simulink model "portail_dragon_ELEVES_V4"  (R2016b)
settings: Solver=VariableStepAuto  StartTime=0.0  StopTime=inf  FixedStep=1e-3  RelTol=1e-3  EnableMultiTasking=on
libraries: fl_lib x6, nesl_utility x5, simulink x2, realtime_pacer_lib x1

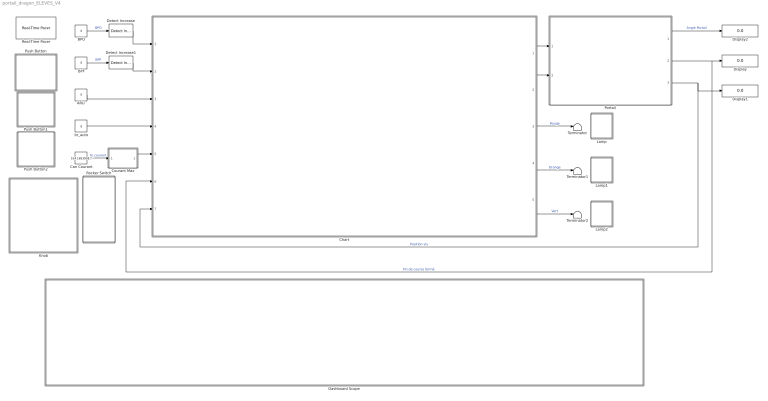
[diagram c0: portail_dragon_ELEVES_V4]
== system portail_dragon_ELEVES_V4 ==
  "ARU " : Constant  Value=0
  BPF : Constant  Value=0
  BPO : Constant  Value=0
  Can Courant : Constant  Value=514.18539581299
  Chart : Stateflow chart  TreatAsAtomicUnit=on
  Courant Max : MATLAB Function  TreatAsAtomicUnit=on
  Dashboard Scope : Subsystem  DialogController=hmiCreateDDGDialog  IsWebBlock=on
  Detect Increase : simulink/Logic and Bit Operations/Detect Increase  vinit=0.0  OutDataTypeStr=boolean
  Detect Increase1 : simulink/Logic and Bit Operations/Detect Increase  vinit=0.0  OutDataTypeStr=boolean
  Display : Display
  Display1 : Display
  Display2 : Display
  Knob : Subsystem  DialogController=hmiCreateDDGDialog  IsWebBlock=on
  Lamp : Subsystem  DialogController=hmiCreateDDGDialog  IsWebBlock=on
  Lamp1 : Subsystem  DialogController=hmiCreateDDGDialog  IsWebBlock=on
  Lamp2 : Subsystem  DialogController=hmiCreateDDGDialog  IsWebBlock=on
  Portail : Subsystem
  Push Button : Subsystem  DialogController=hmiCreateDDGDialog  IsWebBlock=on
  Push Button1 : Subsystem  DialogController=hmiCreateDDGDialog  IsWebBlock=on
  Push Button2 : Subsystem  DialogController=hmiCreateDDGDialog  IsWebBlock=on
  Real-Time Pacer : realtime_pacer_lib/Real-Time Pacer  simTimePerRealTime=1
  Rocker Switch : Subsystem  DialogController=hmiCreateDDGDialog  IsWebBlock=on
  Terminator : Terminator
  Terminator1 : Terminator
  Terminator2 : Terminator
  br_auto : Constant  Value=0
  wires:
  Chart/1(v_mot) -> Portail/1(v_mot)
  Portail/3(pos_vis) -> Chart/7(pos_vis), Display1/1  "Position vis"
  Portail/2(fdc_ferme) -> Display/1, Chart/6(fdc_ferme)  "Fin de course fermé"
  BPO/1 -> Detect Increase/1  "BPO"
  BPF/1 -> Detect Increase1/1  "BPF"
  Portail/1(pos_portail) -> Display2/1  "Angle Portail"
  Can Courant/1 -> Courant Max/1(N_courant)  "N_courant"
  Detect Increase/1 -> Chart/1(bp_ouvrir)
  Detect Increase1/1 -> Chart/2(bp_fermer)
  br_auto/1 -> Chart/4(br_auto)
  Courant Max/1(courant_max) -> Chart/5(courant_max)
  Chart/3(H1) -> Terminator/1  "Rouge"
  Chart/4(H2) -> Terminator1/1  "Orange"
  Chart/5(H3) -> Terminator2/1  "Vert"
  "ARU "/1 -> Chart/3(ARU)
  Chart/2(s_mot) -> Portail/2(s_mot)

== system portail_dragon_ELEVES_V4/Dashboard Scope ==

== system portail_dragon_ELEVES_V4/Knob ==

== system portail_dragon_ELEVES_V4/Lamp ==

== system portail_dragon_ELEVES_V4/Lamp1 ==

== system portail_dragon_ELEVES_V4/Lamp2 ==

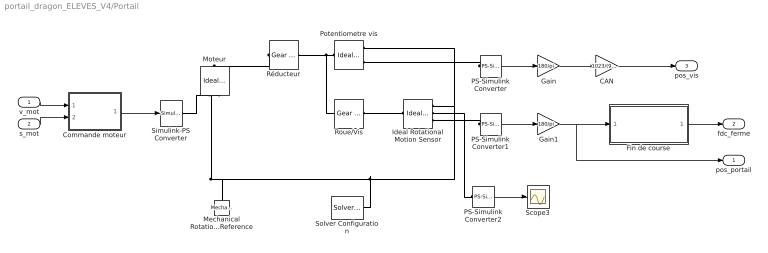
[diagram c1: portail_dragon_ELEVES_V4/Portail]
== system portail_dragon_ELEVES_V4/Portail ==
  v_mot : Inport
  s_mot : Inport  Port=2
  CAN : Gain  Gain=1023/(90*22)
  Commande moteur : MATLAB Function  TreatAsAtomicUnit=on
  Fin de course : MATLAB Function  TreatAsAtomicUnit=on
  Gain : Gain  Gain=180/pi
  Gain1 : Gain  Gain=180/pi
  Ideal Rotational Motion Sensor : fl_lib/Mechanical/Mechanical Sensors/Ideal Rotational Motion Sensor  offset=0 rad
  Mechanical Rotational Reference : fl_lib/Mechanical/Rotational Elements/Mechanical Rotational Reference
  Moteur : fl_lib/Mechanical/Mechanical Sources/Ideal Angular Velocity Source
  PS-Simulink Converter : nesl_utility/PS-Simulink Converter  PhysicalDomain=network_engine_domain  SubClassName=ps_output  LeftPortType=input  RightPortType=output  PseudoPeriodic=off  Frequencies=[]  Unit=1  AffineConversion=off
  PS-Simulink Converter1 : nesl_utility/PS-Simulink Converter  PhysicalDomain=network_engine_domain  SubClassName=ps_output  LeftPortType=input  RightPortType=output  PseudoPeriodic=off  Frequencies=[]  Unit=1  AffineConversion=off
  PS-Simulink Converter2 : nesl_utility/PS-Simulink Converter  PhysicalDomain=network_engine_domain  SubClassName=ps_output  LeftPortType=input  RightPortType=output  PseudoPeriodic=off  Frequencies=[]  Unit=1  AffineConversion=off
  Potentiometre vis : fl_lib/Mechanical/Mechanical Sensors/Ideal Rotational Motion Sensor  offset=0 rad
  Roue/Vis : fl_lib/Mechanical/Mechanisms/Gear Box  ratio=22  t_in_specify=off  t_in_priority=None  t_in=0 N*m  t_out_specify=off  t_out_priority=None  t_out=0 N*m
  Réducteur : fl_lib/Mechanical/Mechanisms/Gear Box  ratio=100  t_in_specify=off  t_in_priority=None  t_in=0 N*m  t_out_specify=off  t_out_priority=None  t_out=0 N*m
  Scope3 : Scope
  Simulink-PS Converter : nesl_utility/Simulink-PS Converter  PhysicalDomain=network_engine_domain  SubClassName=ps_input  LeftPortType=input  RightPortType=output  PseudoPeriodic=off  Frequencies=[]  NoiseDistribution=none  NoiseParameters=[]  Unit=1  AffineConversion=off  InputFiltering=off  SimscapeFilterOrder=1  InputFilterTimeConstant=0.001  UdotUserProvided=1
  Solver Configuration : nesl_utility/Solver Configuration  PhysicalDomain=network_engine_domain  SubClassName=solver  LeftPortType=input  RightPortType=generic  Accelerate=off  Tones=[]  Harmonics=[]  SimulateNoise=off  Profile=off  UseLocalSampling=off  EnableSwitchedLinearOptims=on  FrequencyDomain=off  UseCCode=off  RelTol=0.001  AbsTol=1e-06  MinStep=1e-09  ToWorkspace=off  RevertToSquareIcSolve=off  NumHomotopyIterations=100  PhasorMode=off  PhasorModeNumHarmonics=1  OverrideAbsTol=off  DoDC=off  ResidualTolerance=1e-09  UseLocalSolver=off  LocalSolverChoice=NE_BACKWARD_EULER_ADVANCER  LocalSolverSampleTime=0.001  DoFixedCost=off  MaxNonlinIter=3  MaxModeIter=2  LinearAlgebra=Sparse  DelaysMemoryBudget=1024  AutomaticFiltering=on  FilteringTimeConstant=0.001
  pos_portail : Outport
  fdc_ferme : Outport  Port=2
  pos_vis : Outport  Port=3
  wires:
  Commande moteur/1(wmot) -> Simulink-PS Converter/1
  PS-Simulink Converter/1 -> Gain/1
  Gain1/1 -> pos_portail/1, Fin de course/1(pos_portail)
  Gain/1 -> CAN/1
  v_mot/1 -> Commande moteur/1(v_mot)
  Fin de course/1(fdc_ferme) -> fdc_ferme/1
  PS-Simulink Converter1/1 -> Gain1/1
  CAN/1 -> pos_vis/1
  PS-Simulink Converter2/1 -> Scope3/1
  s_mot/1 -> Commande moteur/2(s_mot)
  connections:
  Réducteur/LConn1 -- Moteur/LConn1
  PS-Simulink Converter1/LConn1 -- Ideal Rotational Motion Sensor/RConn3
  Potentiometre vis/RConn1 -- Solver Configuration/RConn1 -- Moteur/RConn2 -- Mechanical Rotational Reference/LConn1 -- Ideal Rotational Motion Sensor/RConn1
  Simulink-PS Converter/RConn1 -- Moteur/RConn1
  Potentiometre vis/LConn1 -- Roue/Vis/LConn1 -- Réducteur/RConn1
  Ideal Rotational Motion Sensor/LConn1 -- Roue/Vis/RConn1
  PS-Simulink Converter/LConn1 -- Potentiometre vis/RConn3
  PS-Simulink Converter2/LConn1 -- Ideal Rotational Motion Sensor/RConn2

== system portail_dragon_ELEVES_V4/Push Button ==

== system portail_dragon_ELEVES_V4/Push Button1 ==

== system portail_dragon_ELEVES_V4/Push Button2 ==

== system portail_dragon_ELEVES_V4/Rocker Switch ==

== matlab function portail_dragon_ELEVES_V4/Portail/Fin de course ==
function fdc_ferme = fcn(pos_portail)
%#codegen

if pos_portail < 1
    fdc_ferme = 1;
else
    fdc_ferme = 0;
    
end

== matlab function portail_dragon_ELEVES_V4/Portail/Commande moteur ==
function wmot = fcn(v_mot,s_mot)


% Insérer les lignes de codes ci-dessous
wmot = v_mot+s_mot; % à supprimer

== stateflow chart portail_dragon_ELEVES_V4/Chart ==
  state SECU
  state Sens moteur : [group]
    - 0 : Ouvrir
    - 1 : Fermer
  state Fin de course Fermé : [group]
    - 0 : Non fermé
    - 1 : Fermé
  state INIT
  state MANU
    state ATTENTE
    (default) -> ATTENTE
  state AUTO
    state ATTENTE1
    (default) -> ATTENTE1
  INIT -> SECU : after(2,sec)
  SECU -> INIT : after(2,sec)
  (default) -> INIT
  INIT -> (junction 25) : [fdc_ferme==1]
  (junction 25) -> AUTO : [br_auto==1]
  (junction 25) -> MANU : [br_auto==0]
  MANU -> AUTO : [br_auto==1]
  AUTO -> MANU : [br_auto==0]
  data: v_mot output; s_mot output; H1 output; H2 output; H3 output; bp_ouvrir input; bp_fermer input; ARU input; br_auto input; courant_max input; fdc_ferme input; pos_vis input

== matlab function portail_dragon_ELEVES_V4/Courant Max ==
function courant_max = fcn(N_courant)

% Insérer les lignes de codes ci-dessous
courant_max = N_courant; % à supprimer
